(* Logix 5000 AddOnInstructionDefinition export AOI_Remove_Quad_Resolution; software revision 36.00 *)

TYPE DUT_NDSN_spLink_Bead :
STRUCT
   di_rw_NumOfBeads : DINT;
   di_rw_BeadDelay : DINT[8];   // 1/4 mm
   di_rw_BeadDuration : DINT[8];   // 1/4 mm
   di_rw_mode : DINT;   // 1/4 mm
   di_rw_MaxGunTime : DINT;   // microseconds
   di_rw_LineSpeedActivation : DINT;   // 100th m/min
   di_rw_LineSpeedDeactivation : DINT;   // 100th m/min
   di_rw_Interval : DINT;   // 1/4 mm
   di_rw_AdhesiveSavings : DINT;   // 30%-60%
   di_rw_EcoBeadPattern : DINT;   // 0-40, Illegal values: 0,1,11,20,21,30,31,38,39
END_STRUCT
END_TYPE

ADD_ON_INSTRUCTION AOI_Remove_Quad_Resolution   (* revision 1.0 *)
// Raw data from the SpectraLink has a x4 factor included for resolution.  This ADI removes that factor to make editing easier.
VAR_IN_OUT
   Bead_Agg : DUT_NDSN_spLink_Bead; {required}
END_VAR
VAR_INPUT
   i_Counter : INT; {access Read Only}
END_VAR

ROUTINE Logic   (* structured text *)
// Raw data from the SpectraLink has a x4 factor included for resolution.  This ADI removes that factor to make editing easier.
   //
   //
   
   FOR i_Counter := 0 TO 7 DO
   
   	Bead_Agg.di_rw_BeadDelay[i_Counter] := Bead_Agg.di_rw_BeadDelay[i_Counter]/4;
   	Bead_Agg.di_rw_BeadDuration[i_Counter] := Bead_Agg.di_rw_BeadDuration[i_Counter]/4;
   
   END_FOR;
END_ROUTINE
END_ADD_ON_INSTRUCTION
